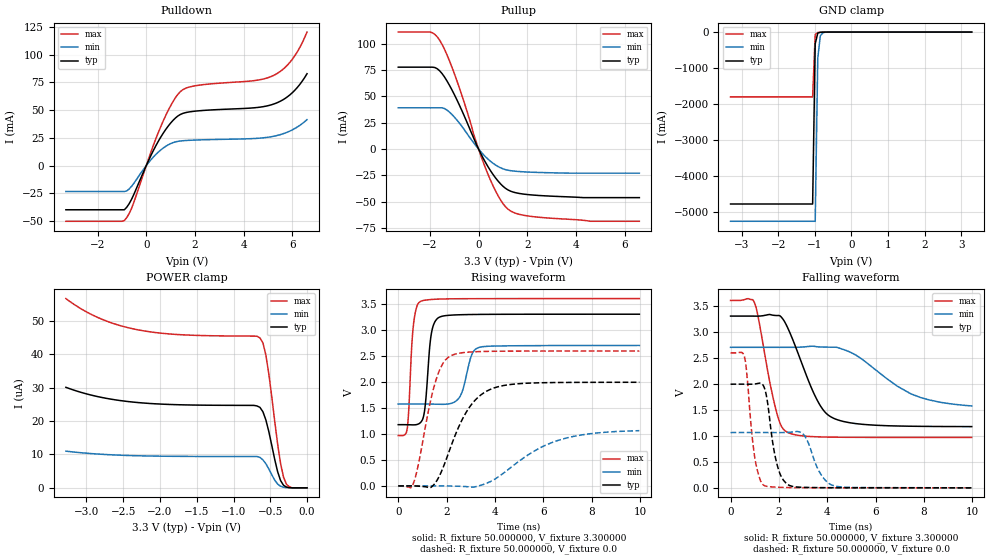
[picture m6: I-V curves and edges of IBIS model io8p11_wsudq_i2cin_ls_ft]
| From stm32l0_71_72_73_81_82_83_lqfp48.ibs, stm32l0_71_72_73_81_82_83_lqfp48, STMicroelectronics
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|   Model io8p11_wsudq_i2cin_ls_ft
[Model]  io8p11_wsudq_i2cin_ls_ft
Model_type I/O
Polarity   Non-Inverting
Enable   Active-Low
Vinl =   0.990000V
Vinh =   2.310000V
Vmeas =  1.650000V
Cref =   50.000000pF
Rref =   100.000000M
Vref =   0.0V
C_comp   3.020400pF   2.988300pF   3.054500pF
[Temperature Range]   25.000000   0.125000k   -40.000000
[Pullup Reference]   3.300000V   2.700000V   3.600000V
[Pulldown Reference]   0.0V   0.0V   0.0V
[POWER Clamp Reference]   3.300000V   2.700000V   3.600000V
[GND Clamp Reference]   0.0V   0.0V   0.0V
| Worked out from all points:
|   slope of the pulldown table from 0 to 0.495 V, typ, clamps not added: 22.6 ohm
|   slope of the pullup table from 0 to 0.495 V, typ, clamps not added: 23.9 ohm
|   GND clamp passes 1 mA (typ) near -0.64 V on its own axis
|   rising waveform, R_fixture 50.000000, V_fixture 3.300000: 20-80 % time 225ps typ, 371ps min, 186ps max; typ from 1.18 V to 3.3 V
|   rising waveform, R_fixture 50.000000, V_fixture 0.0: 20-80 % time 1.18ns typ, 2.2ns min, 710ps max; typ from 0 V to 1.99 V
|   falling waveform, R_fixture 50.000000, V_fixture 3.300000: 20-80 % time 1.13ns typ, 2.07ns min, 655ps max; typ from 3.3 V to 1.18 V
|   falling waveform, R_fixture 50.000000, V_fixture 0.0: 20-80 % time 409ps typ, 576ps min, 329ps max; typ from 1.99 V to 0 V
[Pulldown]
|Voltage   I(typ)   I(min)   I(max)
-3.3V     -39.83mA   -23.37mA   -50.21mA
-900mV    -39.83mA   -23.37mA   -49.53mA
-600mV    -30.28mA   -18.59mA   -38.45mA
500mV     22.11mA    12.28mA    30.1mA
1V        38.33mA    19.81mA    53.88mA
1.4V      46.1mA     22.18mA    66.72mA
2V        49.07mA    23.02mA    71.93mA
4.4V      52.05mA    24.38mA    76.53mA
5.2V      55.25mA    26.31mA    81.02mA
5.6V      59.18mA    28.57mA    86.57mA
6V        65.79mA    32.24mA    95.97mA
6.6V      82.83mA    41.41mA    120.4mA
[Pullup]
|Voltage   I(typ)   I(min)   I(max)
-3.3V     77.63mA    39.16mA    110.9mA
-2V       77.63mA    39.16mA    110.9mA
-1.6V     74.23mA    39.16mA    103.2mA
-1.3V     64.66mA    36.99mA    89.44mA
-900mV    47.13mA    27.82mA    65.37mA
-200mV    10.4mA     5.946mA    13.84mA
300mV     -13.29mA   -7.65mA    -18.99mA
800mV     -30.32mA   -16.54mA   -44.19mA
1.2V      -38.62mA   -20mA      -56.79mA
1.6V      -41.74mA   -21.17mA   -61.39mA
2.5V      -43.99mA   -22.16mA   -64.64mA
6.6V      -46mA      -22.8mA    -68.41mA
[GND_clamp]
|Voltage   I(typ)   I(min)   I(max)
-3.3V     -4.766A    -5.244A    -1.797A
-1.06V    -4.766A    -5.244A    -1.797A
-990mV    -326.6mA   -5.244A    -67.9mA
-920mV    -28.92mA   -722.1mA   -10.96mA
-850mV    -6.612mA   -104.2mA   -6.532mA
-780mV    -3.464mA   -17.27mA   -4.209mA
-500mV    -57.88uA   -167.8uA   -34.02uA
3.28V     0A         0A         0A
[POWER_clamp]
|Voltage   I(typ)   I(min)   I(max)
-3.28V    30.07uA    10.97uA    56.59uA
-2.84V    27.25uA    10.1uA     50.89uA
-2.32V    25.55uA    9.602uA    47.34uA
-640mV    24.06uA    9.099uA    44.84uA
-600mV    22.76uA    8.364uA    43.37uA
-560mV    20.32uA    7.211uA    39.74uA
-520mV    16.86uA    5.675uA    34.14uA
-400mV    4.841uA    1.145uA    13.1uA
-360mV    2.184uA    477.2nA    7.288uA
-320mV    772.4nA    180.3nA    3.213uA
-240mV    60.03nA    0A         295.3nA
0V        0A         0A         0A
[Ramp]
| variable   typ   min   max
dV/dt_r  1.19400/1.18178n   0.61038/2.08043n   1.55532/0.70873n
dV/dt_f  1.27182/1.13117n   0.59214/1.86898n   1.57836/0.65346n
R_load = 50.000000
[Rising Waveform]
R_fixture= 50.000000
V_fixture= 3.300000
V_fixture_min= 2.700000
V_fixture_max= 3.600000
|time   V(typ)   V(min)   V(max)
0s        1.177V     1.573V     968.1mV
360.4ps   1.176V     1.573V     1.067V
620.6ps   1.173V     1.573V     3.056V
920.9ps   1.217V     1.574V     3.546V
1.101ns   1.484V     1.574V     3.569V
1.381ns   2.955V     1.572V     3.583V
1.722ns   3.247V     1.569V     3.591V
2.503ns   3.289V     1.683V     3.597V
3.363ns   3.296V     2.664V     3.599V
9.97ns    3.3V       2.7V       3.6V
[Rising Waveform]
R_fixture= 50.000000
V_fixture= 0.0
V_fixture_min= 0.0
V_fixture_max= 0.0
|time   V(typ)   V(min)   V(max)
0s        -3.187uV   7.689uV    -219.6uV
620.6ps   -717uV     -7.882uV   40.32mV
820.8ps   -5.101mV   3.318uV    384.7mV
1.502ns   38.11mV    180.5uV    1.942V
1.802ns   292.1mV    -173.9uV   2.315V
2.142ns   711.3mV    -2.422mV   2.493V
2.923ns   1.497V     -19.07mV   2.572V
3.944ns   1.88V      116.4mV    2.587V
6.567ns   1.987V     867.7mV    2.592V
9.97ns    1.992V     1.062V     2.593V
[Falling Waveform]
R_fixture= 50.000000
V_fixture= 3.300000
V_fixture_min= 2.700000
V_fixture_max= 3.600000
|time   V(typ)   V(min)   V(max)
0s        3.3V       2.7V       3.6V
981ps     3.3V       2.7V       3.564V
1.862ns   3.312V     2.7V       1.527V
2.082ns   3.289V     2.7V       1.202V
2.322ns   3.114V     2.7V       1.075V
3.483ns   1.776V     2.717V     981.8mV
4.124ns   1.37V      2.703V     974.3mV
5.165ns   1.235V     2.555V     970.2mV
7.467ns   1.184V     1.804V     968.4mV
9.97ns    1.177V     1.573V     968.1mV
[Falling Waveform]
R_fixture= 50.000000
V_fixture= 0.0
V_fixture_min= 0.0
V_fixture_max= 0.0
|time   V(typ)   V(min)   V(max)
0s        1.992V     1.062V     2.593V
580.6ps   1.992V     1.062V     2.51V
1.001ns   1.995V     1.062V     585.8mV
1.381ns   1.94V      1.062V     47.02mV
1.922ns   450.2mV    1.061V     12.15mV
2.442ns   44.27mV    1.068V     4.959mV
3.043ns   8.868mV    1.011V     2.135mV
3.724ns   3.746mV    267.2mV    1.112mV
4.324ns   2.243mV    34.55mV    630.3uV
9.97ns    -3.187uV   7.689uV    -219.6uV
